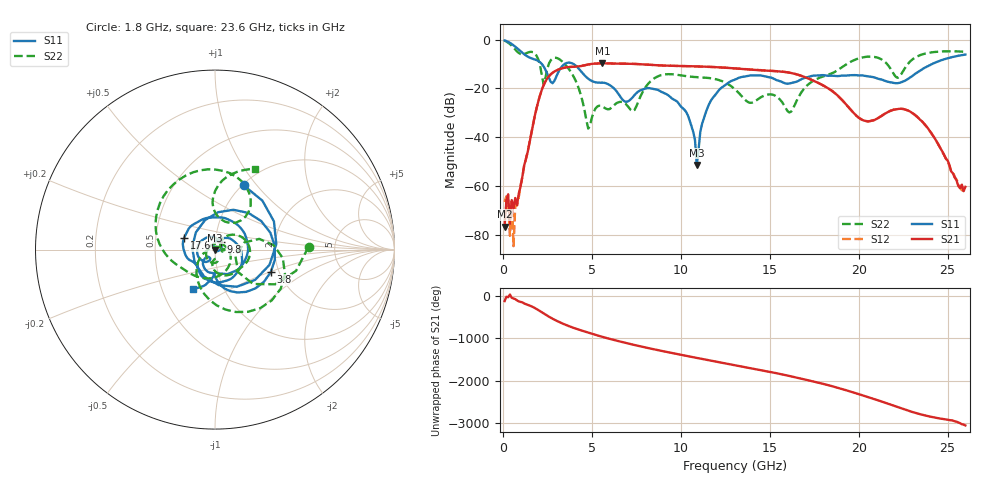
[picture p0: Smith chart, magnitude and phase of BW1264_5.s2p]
!Keysight Technologies,N5245B,MY57181159,A.13.60.06
!Date: Friday, December 18, 2020 23:52:11
!Correction: S11(Full 2 Port(1,2))
!S21(Full 2 Port(1,2))
!S12(Full 2 Port(1,2))
!S22(Full 2 Port(1,2))
!S2P File: Measurements: S11, S21, S12, S22:
# Hz S  dB  R 50
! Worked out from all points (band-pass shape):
!   260 points, 100 MHz to 26 GHz, reference 50 ohm
!   highest |S21| = -9.72 dB at 5.6 GHz (marker M1); lowest = -76.6 dB at 100 MHz (marker M2)
!   |S21| within 3 dB of the highest: 2.984 GHz to 14.84 GHz (11.85 GHz wide, 133 % of centre)
!   lowest |S11| = -51.3 dB at 10.9 GHz (marker M3), VSWR 1.01, Z = 50 - j0.269 ohm
!   |S11| at or under -10 dB: 2.196 GHz to 3.47 GHz (1.274 GHz wide, 45 % of centre); 3.971 GHz to 24.12 GHz (20.15 GHz wide, 143 % of centre)
!   |S22| runs from -36.5 to -0.4 dB; largest |S21 - S12| = 0.00058
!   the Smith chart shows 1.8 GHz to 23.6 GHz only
!   S11 on the Smith chart (normalised r, x): 1.8 GHz: 1.02, +0.86; 3.8 GHz: 1.81, -0.51; 9.8 GHz: 1.06, +0.09; 17.6 GHz: 0.70, +0.09; 23.6 GHz: 0.72, -0.34
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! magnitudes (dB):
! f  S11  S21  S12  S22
! 100 MHz  -0.3  -76.6  -66.6  -0.4
! 300 MHz  -0.9  -63.4  -68.3  -1.3
! 400 MHz  -1.3  -75.5  -80.4  -1.8
! 500 MHz  -1.8  -65.8  -66.2  -2.5
! 600 MHz  -2.3  -69.1  -84.7  -3.2
! 1.8 GHz  -8.1  -31.1  -31.2  -5.7
! 2.3 GHz  -11.1  -18.6  -18.6  -18.6
! 3.8 GHz  -9.5  -11.2  -11.2  -13.0
! 4.5 GHz  -13.9  -10.7  -10.7  -25.9
! 4.8 GHz  -16.0  -10.2  -10.2  -36.5
! 5.6 GHz  -17.6  -9.7  -9.7  -27.4
! 8.8 GHz  -20.9  -10.6  -10.5  -14.8
! 9.8 GHz  -25.4  -10.8  -10.8  -14.4
! 10.9 GHz  -51.3  -11.0  -11.0  -15.4
! 11.6 GHz  -26.3  -11.1  -11.1  -15.7
! 13.1 GHz  -16.2  -11.8  -11.8  -20.7
! 16.1 GHz  -18.0  -13.5  -13.5  -29.9
! 17.4 GHz  -14.8  -16.6  -16.6  -17.1
! 17.6 GHz  -14.7  -17.3  -17.3  -16.3
! 21.7 GHz  -17.4  -29.5  -29.5  -10.9
! 23.6 GHz  -12.0  -33.8  -33.8  -6.0
! 26 GHz  -6.1  -60.4  -61.0  -5.0
